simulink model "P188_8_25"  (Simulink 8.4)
settings: Solver=ode45  StartTime=0.0  StopTime=10.0  RelTol=1e-3
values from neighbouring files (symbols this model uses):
  k = k+1    (= 2)    [while_break.m]    (also in FurikoSlvCheck.m = 0.2)

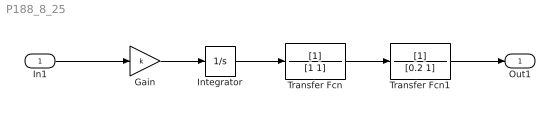
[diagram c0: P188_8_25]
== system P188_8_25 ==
  In1 : Inport
  Gain : Gain  Gain=k
  Integrator : Integrator
  Transfer Fcn : TransferFcn  Denominator=[1 1]
  Transfer Fcn1 : TransferFcn  Denominator=[0.2 1]
  Out1 : Outport
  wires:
  Integrator/1 -> Transfer Fcn/1
  Transfer Fcn/1 -> Transfer Fcn1/1
  Gain/1 -> Integrator/1
  Transfer Fcn1/1 -> Out1/1
  In1/1 -> Gain/1
